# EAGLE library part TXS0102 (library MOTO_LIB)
2-BIT BIDIRECTIONAL VOLTAGE-LEVEL TRANSLATOR FOR OPEN-DRAIN AND PUSH-PULL APPLICATIONS
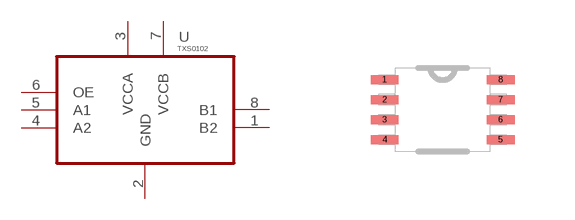
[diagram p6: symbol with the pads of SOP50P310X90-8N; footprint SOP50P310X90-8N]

Designator prefix U

## TXS0102 (MPN: TXS0102DCUR; SUPPLIER: TEXAS INSTRUMENTS)  [SOP50P310X90-8N]
1  B2
2  GND  pas
3  VCCA  pwr
4  A2
5  A1
6  OE  in
7  VCCB  pwr
8  B1

## Footprint SOP50P310X90-8N (pad centres in mm)
smd 0.7 x 0.23: 1 -1.45,0.75; 2 -1.45,0.25; 3 -1.45,-0.25; 4 -1.45,-0.75; 5 1.45,-0.75; 6 1.45,-0.25; 7 1.45,0.25; 8 1.45,0.75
